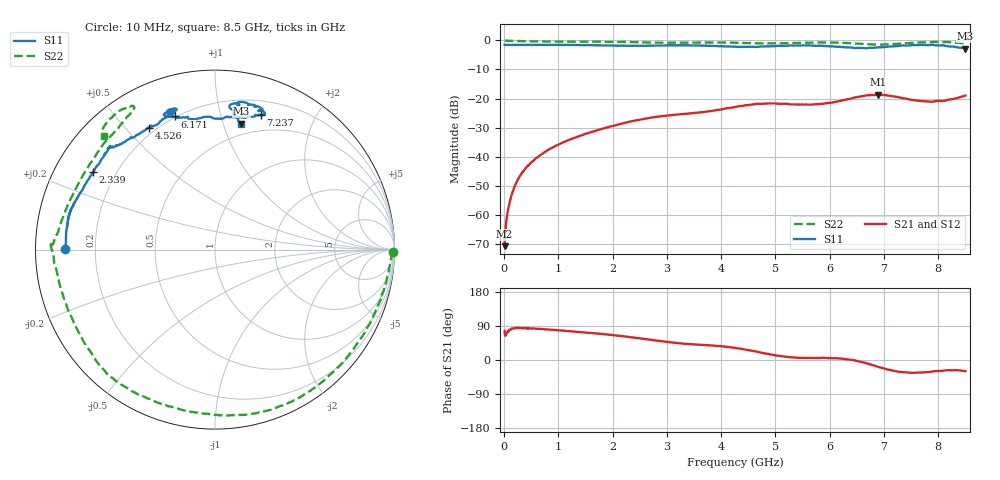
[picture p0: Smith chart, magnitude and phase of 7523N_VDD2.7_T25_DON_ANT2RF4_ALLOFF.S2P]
!Agilent Technologies,E5071C,MY46417908,A.11.23
!Date: Wed Dec 09 17:50:34 2020
!Data & Calibration Information:
!Freq	S11:SOLT2(ON)	S21:SOLT2(ON)	S12:SOLT2(ON)	S22:SOLT2(ON)
!PortZ  Port1:50+j0  Port2:50+j0
!Above PortZ is port z conversion or system Z0 setting when saving the data.
!When reading, reference impedance value at option line is always used.
# Hz S dB R 50
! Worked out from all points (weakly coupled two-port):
!   1601 points, 10 MHz to 8.5 GHz, reference 50 ohm
!   highest |S21| = -18.70 dB at 6.898 GHz (marker M1); lowest = -70.7 dB at 10 MHz (marker M2)
!   lowest |S11| = -2.9 dB at 8.5 GHz (marker M3), VSWR 6.06, Z = 19.9 + j57.4 ohm
!   |S11| at or under -10 dB: nowhere
!   |S22| runs from -1.5 to 0.0 dB; largest |S21 - S12| = 0.0012
!   S11 on the Smith chart (normalised r, x): 10 MHz: 0.09, +0.00; 2.339 GHz: 0.12, +0.29; 4.526 GHz: 0.17, +0.58; 6.171 GHz: 0.20, +0.73; 7.237 GHz: 0.34, +1.34; 8.5 GHz: 0.40, +1.15
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1e7  -1.57 179.7  -70.69 76.8  -69.58 72.7  -0.05 -0.9
7.3675e7  -1.59 178.6  -58.17 75.9  -58.20 76.6  -0.15 -3.0
1.3735e8  -1.59 177.5  -53.14 82.1  -53.19 82.0  -0.19 -5.1
2.328625e8  -1.59 175.8  -48.62 84.3  -48.65 84.4  -0.24 -8.3
3.602125e8  -1.57 173.6  -44.94 83.8  -44.94 83.7  -0.30 -12.7
8.112438e8  -1.56 167.8  -37.68 80.7  -37.67 80.8  -0.42 -29.8
1.426769e9  -1.65 162.9  -32.59 73.4  -32.59 73.3  -0.46 -54.5
2.339444e9  -1.89 147.6  -27.83 60.1  -27.83 60.0  -0.60 -81.0
2.843538e9  -1.80 138.4  -26.19 50.6  -26.17 50.6  -0.78 -98.5
3.459062e9  -1.77 135.7  -25.03 41.7  -25.02 41.6  -0.78 -120.3
4.255e9  -2.16 126.8  -22.92 32.1  -22.91 32.0  -0.83 -135.6
4.525619e9  -2.25 118.4  -22.17 25.4  -22.16 25.3  -0.96 -143.5
5.289719e9  -1.75 107.1  -22.01 7.5  -22.03 7.6  -0.93 -175.9
5.671769e9  -1.83 108.8  -22.07 5.2  -22.05 5.7  -0.79 178.3
6.170556e9  -2.22 106.7  -20.90 4.2  -20.95 4.3  -0.84 178.2
6.520769e9  -2.60 94.7  -19.45 -3.3  -19.50 -3.3  -1.14 172.5
6.897512e9  -2.49 78.8  -18.70 -18.2  -18.72 -18.1  -1.47 150.9
7.088538e9  -2.12 73.4  -18.98 -25.6  -19.04 -25.6  -1.37 137.4
7.237112e9  -2.03 71.1  -19.42 -30.0  -19.41 -30.1  -1.26 128.5
7.719981e9  -1.59 76.0  -20.90 -32.4  -20.88 -32.4  -0.66 120.1
8.139175e9  -1.93 84.2  -20.63 -27.1  -20.63 -27.0  -0.59 129.0
8.5e9  -2.89 78.3  -18.97 -29.3  -18.95 -28.9  -1.08 134.3
